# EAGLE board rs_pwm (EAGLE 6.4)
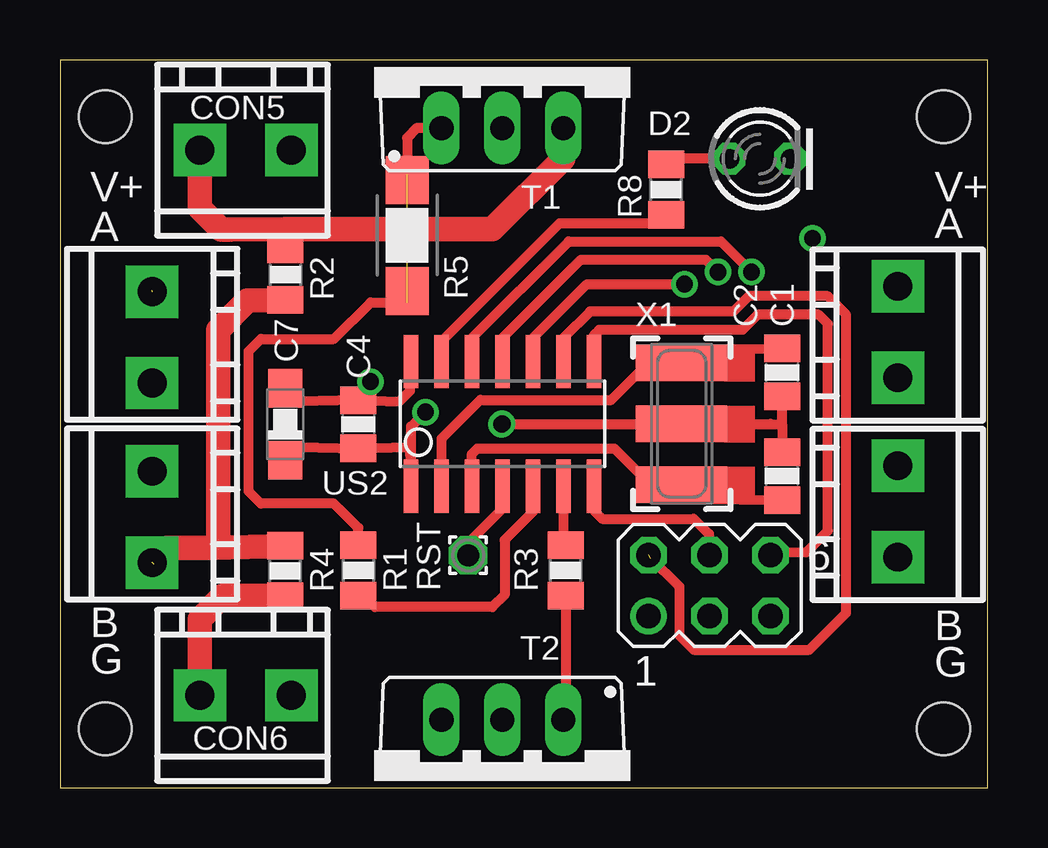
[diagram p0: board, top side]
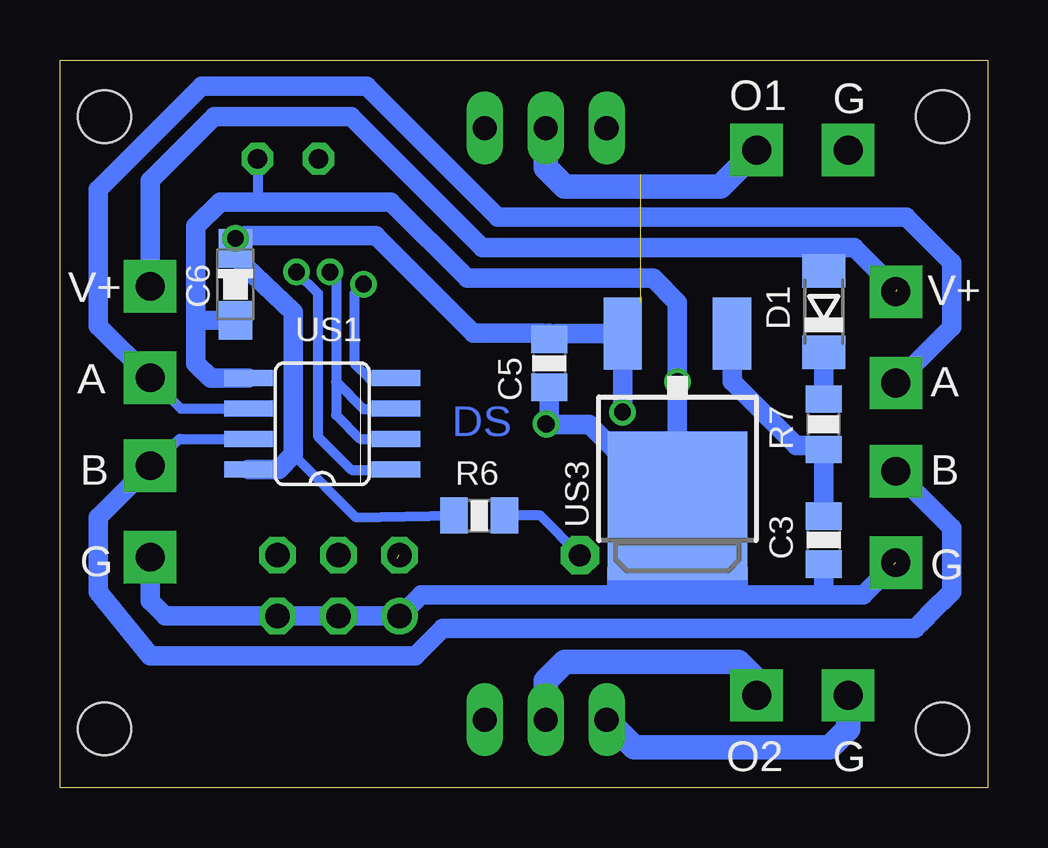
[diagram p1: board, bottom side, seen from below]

Size 38.67 x 30.33 mm. Coordinates in mm from the lower left corner, seen from the top.
Outline: 0,0 38.67,0 38.67,30.33 0,30.33 0,0
Copper layers (1*16): Top 0.035mm / dielectric 1.5mm / Bottom 0.035mm
Design rules "default": minimum track width 10mil, minimum drill 24mil, track to track 8mil, track to pad 8mil, pad to pad 8mil, via to via 8mil, smd to smd 8mil, copper to edge 40mil, drill to drill 8mil, minimum pad ring 10mil, minimum via ring 8mil, stop-mask expansion 4mil, vias tented up to drill 0mil, thermal gap 10mil
Holes 2.2 mm at 1.89,27.97 1.89,2.45 36.82,2.45 36.82,27.97

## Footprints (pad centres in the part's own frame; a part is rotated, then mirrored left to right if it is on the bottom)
C0805 = smd 1.143 x 1.5: 1 -1.001,0; 2 1.001,0
SMC_A = smd 1.6 x 1.4: + -1.5,0; - 1.5,0
ARK2/300 = drill 1.2 pad 2.184 square: 1 -2.54,0; 2 1.27,0
SOD80C = smd 1.4 x 1.8: A 1.7,0; C -1.7,0
LED3MM = drill 0.813 octagon: A -1.27,0; K 1.27,0
MA03-2 = drill 1.016: 1 -2.54,-1.27 | drill 1.016 octagon: 2 -2.54,1.27; 3 0,-1.27; 4 0,1.27; 5 2.54,-1.27; 6 2.54,1.27
R0805 = smd 1.143 x 1.5: 1 -1.052,0; 2 1.052,0
R2010W = smd 2 x 1.8: 1 -2.311,0; 2 2.311,0
1,6/0,9 = drill 0.914 pad 1.6 octagon: 1 0,0
TO220BV = drill 1.016 long: D 0,-2.54; G -2.54,-2.54; S 2.54,-2.54
SO08 = smd 0.66 x 2.032: 1 -1.905,-3.073; 2 -0.635,-3.073; 3 0.635,-3.073; 4 1.905,-3.073; 5 1.905,3.073; 6 0.635,3.073; 7 -0.635,3.073; 8 -1.905,3.073
SOIC14 = smd 0.61 x 2.21: 1 -3.81,-2.603; 2 -2.54,-2.603; 3 -1.27,-2.603; 4 0,-2.603; 5 1.27,-2.603; 6 2.54,-2.603; 7 3.81,-2.603; 8 3.81,2.603; 9 2.54,2.603; 10 1.27,2.603; 11 0,2.603; 12 -1.27,2.603; 13 -2.54,2.603; 14 -3.81,2.603
DPACK = smd 1.6 x 3: 1 -2.28,-4.8; 3 2.28,-4.8 | smd 5.8 x 6.2: 4 0,2.38
Q4M_SMD = smd 1.524 x 3.81: 1 -2.54,0; 2 0,0; 3 2.54,0

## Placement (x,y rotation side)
C1  18pF  [C0805]  30.08,17.3 270 top
C2  18pF  [C0805]  30.08,12.99 90 top
C3  100nF  [C0805]  6.84,10.32 270 bottom
C4  100nF  [C0805]  12.43,15.15 90 top
C5  100nF  [C0805]  18.27,17.69 270 bottom
C6  1uF  [SMC_A]  31.36,20.99 270 bottom
C7  1uF  [SMC_A]  9.38,15.15 90 top
CON1  [ARK2/300]  3.84,18.13 270 top
CON2  [ARK2/300]  34.91,19.63 90 top
CON3  [ARK2/300]  3.84,10.65 270 top
CON4  [ARK2/300]  34.91,12.15 90 top
CON5  [ARK2/300]  8.37,26.58 0 top
CON6  [ARK2/300]  8.37,3.84 0 top
D1  4148  [SOD80C]  6.84,19.84 90 bottom
D2  [LED3MM]  29.16,26.22 0 top
PROG  [MA03-2]  27.07,8.42 0 top
R1  2k  [R0805]  12.43,9.05 270 top
R2  22R  [R0805]  9.39,21.38 270 top
R3  2k  [R0805]  21.07,9.05 90 top
R4  22R  [R0805]  9.38,9.03 90 top
R5  [R2010W]  14.46,23.02 90 top
R6  2k  [R0805]  21.2,11.34 0 bottom
R7  22R  [R0805]  6.84,15.15 270 bottom
R8  2k  [R0805]  25.26,24.93 270 top
RST  [1,6/0,9]  17,9.69 0 top
T1  BUZ11BV  [TO220BV]  18.43,30.03 0 top
T2  BUZ11BV  [TO220BV]  18.43,0.29 180 top
US1  MAX485  [SO08]  27.74,15.17 90 bottom
US2  TINY24/44/84-SSU  [SOIC14]  18.44,15.17 0 top
US3  78M05  [DPACK]  12.94,14.13 180 bottom
X1  12MHz  [Q4M_SMD]  25.9,15.17 270 top

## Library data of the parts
C1-C7 R1-R8 = rcl
CON1-CON6 = ds_lib_eagle
D1 = diode
D2 = led
PROG = con-lstb; OC_FARNELL: unknown; OC_NEWARK: unknown
RST = wirepad
T1 T2 = transistor-power
US1 = maxim; MF: MAXIM; MPN: MAX481CSA; OC_FARNELL: unknown; OC_NEWARK: 90C3817
US2 = avr-4
US3 = v-reg
X1 = DS

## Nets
GND: C1.2 C2.2 C3.2 C4.2 C5.2 C6.- C7.- CON3.2 CON4.1 D2.K PROG.1 PROG.3 PROG.5 R2.2 R4.2 US1.5 US2.14 US3.4 X1.2
L_A: CON1.2 CON2.1 US1.6
L_B: CON3.1 CON4.2 US1.7
LED: R8.2 US2.13
MISO: PROG.6 US2.8
MOSI: PROG.4 US2.7
N$1: D2.A R8.1
N$2: R1.1 T1.G
N$3: R3.1 T2.G
N$4: CON5.2 T1.D
N$5: D1.C R7.1
N$6: CON5.1 R2.1 T1.S
N$7: CON6.1 R4.1 T2.S
N$8: CON6.2 T2.D
N$9: C3.1 R7.2 US3.1
RST: R6.2 RST.1 US2.4
RXD: US1.1 US2.12
SCK: PROG.2 US2.9
SIG1: R3.2 US2.6
SIG2: R1.2 US2.5
TEN: US1.2 US1.3 US2.11
TXD: US1.4 US2.10
V+: CON1.1 CON2.2 D1.A
VDD: C4.1 C5.1 C6.+ C7.+ R6.1 US1.8 US2.1 US3.3
X1: C1.1 US2.2 X1.1
X2: C2.1 US2.3 X1.3

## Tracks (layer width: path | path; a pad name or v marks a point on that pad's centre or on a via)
GND  (via drill 0.7)  (1 unrouted)
  Top 0.406: C4.2 14.14,16.1 14.59,16.54 14.59,17.74 US2.14 | C4.2 9.93,16.1 C7.- | 30.08,15.15 C2.2 | 30.08,15.15 C1.2 | 30.08,15.15 29.6,15.17 X1.2 v18.42,15.17 v18.4,15.15 | C4.2 12.94,16.42 v12.94,16.92
  Top 1.016: R4.2 6.34,9.98 | 6.34,9.98 4.44,9.98 CON3.2 | R2.2 7.81,20.3 6.59,19.08 6.59,10.24 6.34,9.98
  Bottom 0.406: CON4.1 34.58,9.94 | D2.K 30.43,24.64 30.21,24.42
  Bottom 0.813: CON4.1 34.91,7.78 34.28,7.15 PROG.5 PROG.3 PROG.1 24.49,7.15 23.61,8.03 13.07,8.03 | v18.42,15.17 18.29,15.17 18.27,15.15 | US3.4 12.94,12.35 | 12.94,12.35 v12.94,16.92 | v12.94,16.92 12.94,20.23 13.96,21.24 21.7,21.24 24.88,24.42 30.21,24.42 31.99,24.42 33.01,23.4 33.01,19.46 | 18.27,15.15 C5.2 | 18.27,15.15 16.62,15.15 14.85,13.37 13.96,13.37 12.94,12.35 | C6.- 31.89,19.49 33.01,19.46 | US1.5 32.39,17.07 33.01,17.69 33.01,19.46 | CON3.2 3.85,9.38 | 13.07,8.03 6.84,8.03 | 6.84,8.03 5.19,8.03 3.92,9.3 | C3.2 6.84,8.03 | v12.94,16.92 12.94,8.16 13.07,8.03
L_A
  Bottom 0.406: US1.6 33.63,15.8 CON2.1
  Bottom 0.813: 3.6,17.12 CON1.2 1.51,19.19 1.51,21.88 3.41,23.78 20.43,23.78 25.89,29.24 32.75,29.24 37.07,24.93 37.07,19.25 CON2.1
L_B
  Bottom 0.406: US1.7 33.67,14.53 CON4.2
  Bottom 0.813: CON3.1 3.84,13.16 1.51,10.83 1.51,8.16 2.4,7.27 2.65,7.02 2.78,6.89 3.03,6.64 22.72,6.64 23.86,5.49 34.91,5.49 37.07,8.16 37.07,11.26 CON4.2
LED
  Top 0.406: US2.13 15.9,18.61 20.81,23.53 24.81,23.53 R8.2
MISO
  Top 0.406: US2.8 22.25,18.86 22.46,19.08 28.43,19.08 29.07,19.72 31.61,19.72 31.99,19.34 31.99,10.7 31.1,9.81 29.7,9.82 PROG.6
MOSI
  Top 0.406: US2.7 22.25,11.55 22.59,11.21 26.4,11.21 27.04,10.57 27.04,10.04 PROG.4
N$1
  Top 0.406: D2.A 25.35,26.22 R8.1
N$2  (1 unrouted)
  Top 0.406: T1.G 14.87,27.49 14.46,27.08 14.46,25.56 | R1.1 12.43,10.83 11.42,11.84 8.37,11.84 7.86,12.35 7.86,18.19 8.37,18.7 11.42,18.7 12.94,20.23 14.46,20.23
N$3
  Top 0.406: R3.1 21.07,3.69 T2.G
N$4
  Bottom 1.016: T1.D 18.43,25.84 17.64,25.05 11.16,25.05 CON5.2
N$5
  Bottom 0.813: R7.1 D1.C
N$6
  Top 1.016: R2.1 9.39,23.27 | 9.39,23.27 7.1,23.27 6.72,23.27 5.83,24.16 CON5.1 | T1.S 20.97,26.22 18.02,23.27 9.39,23.27
N$7
  Top 1.016: R4.1 6.79,7.98 5.83,7.02 CON6.1
  Bottom 1.016: CON6.1 5.83,2.45 6.59,1.68 14.74,1.68 T2.S
N$8
  Bottom 1.016: T2.D 18.43,4.45 17.64,5.24 10.4,5.24 9.64,4.48 CON6.2
N$9
  Bottom 0.813: C3.1 R7.2 7.16,14.26 7.99,14.26 10.66,16.93 US3.1
RST
  Top 0.406: US2.4 18.44,11.62 17,10.19 RST.1
  Bottom 0.406: RST.1 18.65,11.34 R6.2
RXD  (via drill 0.7)
  Top 0.406: US2.12 17.17,18.74 21.2,22.77 27.54,22.77 v28.82,21.5
  Bottom 0.406: v28.82,21.5 27.93,20.61 27.93,14.64 26.53,13.24 24.69,13.24 US1.1
SCK  (1 unrouted)
  Top 0.406: US2.9 20.98,18.74 22.08,19.84 28.05,19.84 28.69,20.48 31.99,20.48 32.75,19.72 32.75,7.27 31.23,5.75 26.4,5.75 25.8,6.35 25.8,8.38 24.62,9.56
SIG1
  Top 0.406: US2.6 20.98,10.22 R3.2
SIG2
  Top 0.406: US2.5 19.71,11.5 18.53,10.32 18.53,8.03 18.02,7.53 13.13,7.53 R1.2
TEN  (via drill 0.7)
  Top 0.406: US2.11 18.44,18.74 21.7,22 26.91,22 v27.42,21.5
  Bottom 0.406: v27.42,21.5 27.16,21.24 27.16,16.92 | 27.16,16.92 26.02,15.78 24.69,15.78 US1.3 | US1.2 26.17,14.53 27.16,15.53 27.16,16.92
TXD  (via drill 0.7)
  Top 0.406: US2.10 19.71,18.74 21.96,20.99 v26.02,20.99
  Bottom 0.406: v26.02,20.99 26.4,20.61 26.4,17.69 25.77,17.05 24.56,17.05 US1.4
V+  (1 unrouted)
  Bottom 0.813: CON2.2 34.91,25.31 32.24,27.97 26.53,27.97 21.07,22.51 6.97,22.51 | 6.97,22.51 5.57,22.51 3.8,20.73 | D1.A 7.1,21.88 7.1,22.38 6.97,22.51
VDD  (via drill 0.7)
  Top 0.406: 9.26,13.52 C7.+ 9.93,14.2 C4.1 14.53,14.2 14.59,13.88 14.59,12.6 US2.1 14.63,15.05 v15.23,15.65
  Bottom 0.406: US3.3 | R6.1 26.34,11.27 28.94,13.88 | v31.36,22.89 31.1,22.13 31.36,22.38
  Bottom 0.813: v15.23,15.65 US3.3 | US3.3 17.98,18.93 C5.1 | C5.1 18.27,18.96 | US1.8 29.56,13.26 28.94,13.88 28.94,19.82 30.97,21.75 31.36,22.13 31.36,22.38 C6.+ 31.61,22.64 31.36,22.64 30.97,23.02 25.51,23.02 21.45,18.96 18.59,18.96 C5.1
X1
  Top 0.406: US2.2 15.9,14.55 17.51,16.16 22.97,16.16 24.62,17.81 25.13,17.81 | 25.13,17.81 25.8,17.81 X1.1 | C1.1 25.57,18.26 25.13,17.81
X2
  Top 0.406: US2.3 17.17,13.91 17.39,14.13 23.1,14.13 24.5,12.73 25.8,12.73 X1.3 26.49,12.04 C2.1
(copper drawn outside any net)
  shapes: Bottom area x1, Top area x3

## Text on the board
Bottom: DS
tPlace: V+ | V+ | A | A | RST | B | B | G | G
bPlace: G | O1 | V+ | V+ | A | A | B | B | G | G | G | O2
